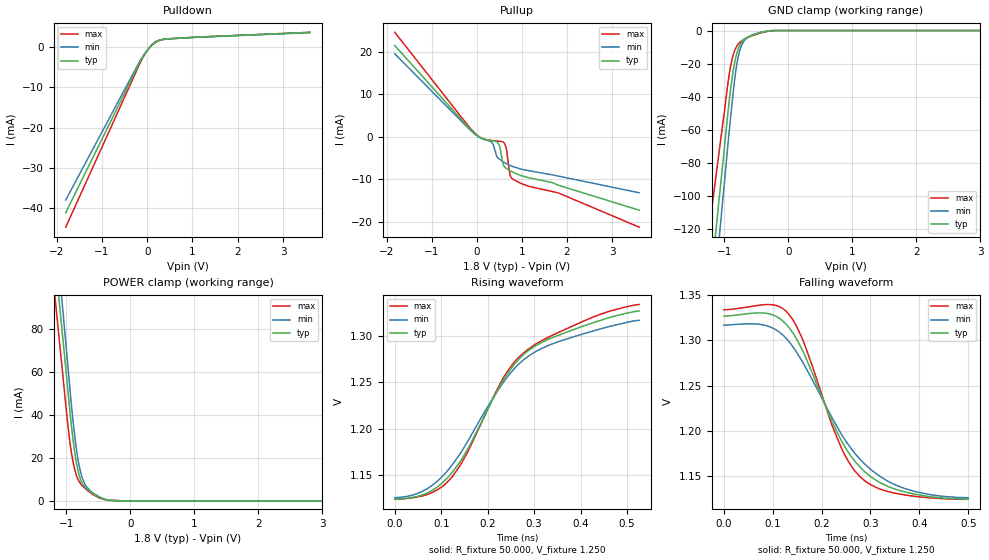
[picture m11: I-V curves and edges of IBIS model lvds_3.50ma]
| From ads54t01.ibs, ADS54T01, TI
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[Model]   lvds_3.50ma
Model_type 3-state
Vref=1.250E+00
Rref=5.000E+01
Cref=0.000E+00
Vmeas=1.250E+00
C_comp   7.860E-13   7.790E-13   7.930E-13
[Voltage Range]   1.800E+00   1.650E+00   1.950E+00
[POWER Clamp Reference]   1.800E+00   1.650E+00   1.950E+00
[GND Clamp Reference]   0.000E+00   0.000E+00   0.000E+00
[Pullup Reference]   1.800E+00   1.650E+00   1.950E+00
[Pulldown Reference]   0.000E+00   0.000E+00   0.000E+00
[Temperature Range]   25   85   -40
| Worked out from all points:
|   slope of the pulldown table from 0 to 0.27 V, typ, clamps not added: 106 ohm
|   slope of the pullup table from 0 to 0.27 V, typ, clamps not added: 231 ohm
|   GND clamp passes 1 mA (typ) near -0.41 V on its own axis
|   POWER clamp passes 1 mA (typ) near -0.41 V on its own axis
|   rising waveform, R_fixture 50.000, V_fixture 1.250: 20-80 % time 153ps typ, 161ps min, 159ps max; typ from 1.12 V to 1.33 V
|   falling waveform, R_fixture 50.000, V_fixture 1.250: 20-80 % time 107ps typ, 128ps min, 87.4ps max; typ from 1.33 V to 1.12 V
[GND Clamp]
-1.8V     -374.4mA   -423.5mA   -288.4mA
-1.02V    -78.69mA   -100.5mA   -54.92mA
-920mV    -41.17mA   -59.34mA   -25.51mA
-860mV    -23.88mA   -36.88mA   -14.48mA
-820mV    -15.94mA   -23.97mA   -10.43mA
-780mV    -10.76mA   -15.27mA   -8.038mA
-740mV    -7.589mA   -9.923mA   -6.562mA
-700mV    -5.657mA   -6.755mA   -5.499mA
-640mV    -4.069mA   -4.329mA   -4.359mA
-460mV    -1.489mA   -1.354mA   -1.806mA
-220mV    -4.201uA   -14.01uA   -11.29uA
3.6V      0A         0A         0A
[Power Clamp]
-1.8V     302.8mA    334.3mA    279.3mA
-1.76V    290.6mA    320.1mA    266.6mA
-1.06V    77.25mA    90.47mA    60.21mA
-940mV    40.5mA     50.88mA    26.54mA
-880mV    24.97mA    33.1mA     16.1mA
-820mV    14.43mA    19.78mA    10.24mA
-780mV    10.23mA    13.83mA    8.195mA
-720mV    6.913mA    8.542mA    6.262mA
-580mV    3.451mA    3.702mA    2.982mA
-360mV    441.4uA    538.8uA    356.5uA
-140mV    0A         9.789uA    18.55uA
3.6V      0A         0A         0A
[Pullup]
-1.82V    21.53mA    19.59mA    24.65mA
-20mV     503.5uA    417.8uA    616.9uA
320mV     -908.4uA   -1.137mA   -845.2uA
460mV     -1.285mA   -4.895mA   -1.001mA
500mV     -2.059mA   -5.283mA   -1.043mA
600mV     -6.864mA   -5.979mA   -1.351mA
660mV     -7.486mA   -6.339mA   -3.134mA
740mV     -8.005mA   -6.751mA   -9.101mA
780mV     -8.235mA   -6.928mA   -9.819mA
1.16V     -9.671mA   -8.003mA   -11.7mA
1.8V      -11.39mA   -9.245mA   -13.2mA
3.6V      -17.3mA    -13.19mA   -21.3mA
[Pulldown]
-1.8V     -41.19mA   -38.04mA   -44.8mA
-160mV    -3.661mA   -3.394mA   -3.982mA
-40mV     -1.393mA   -1.319mA   -1.477mA
80mV      280.2uA    222.4uA    370uA
180mV     1.229mA    1.13mA     1.348mA
320mV     1.869mA    1.817mA    1.894mA
520mV     2.132mA    2.128mA    2.101mA
3.6V      3.683mA    3.624mA    3.702mA
[Rising Waveform]
R_fixture = 50.000
V_fixture = 1.250
V_fixture_min = 1.250
V_fixture_max = 1.250
|  time   V(typ)   V(min)   V(max)
0s        1.124V     1.126V     1.124V
66ps      1.13V      1.134V     1.129V
120ps     1.151V     1.159V     1.146V
156ps     1.177V     1.186V     1.174V
232ps     1.251V     1.249V     1.254V
256ps     1.269V     1.264V     1.271V
288ps     1.284V     1.278V     1.286V
338ps     1.298V     1.291V     1.3V
426ps     1.314V     1.305V     1.32V
526ps     1.327V     1.317V     1.334V
[Falling Waveform]
R_fixture = 50.000
V_fixture = 1.250
V_fixture_min = 1.250
V_fixture_max = 1.250
|  time   V(typ)   V(min)   V(max)
0s        1.327V     1.317V     1.334V
88ps      1.33V      1.316V     1.34V
134ps     1.314V     1.298V     1.328V
164ps     1.286V     1.273V     1.297V
218ps     1.214V     1.218V     1.211V
242ps     1.187V     1.195V     1.179V
266ps     1.168V     1.176V     1.157V
288ps     1.155V     1.163V     1.145V
370ps     1.132V     1.136V     1.129V
500ps     1.124V     1.126V     1.124V
[Ramp]
dV/dt_r   1.1216E-01/1.5250E-10   1.1472E-01/1.6090E-10   1.2606E-01/1.5850E-10
dV/dt_f   1.1216E-01/1.0691E-10   1.1472E-01/1.2806E-10   1.2606E-01/8.7078E-11
R_load = 50
